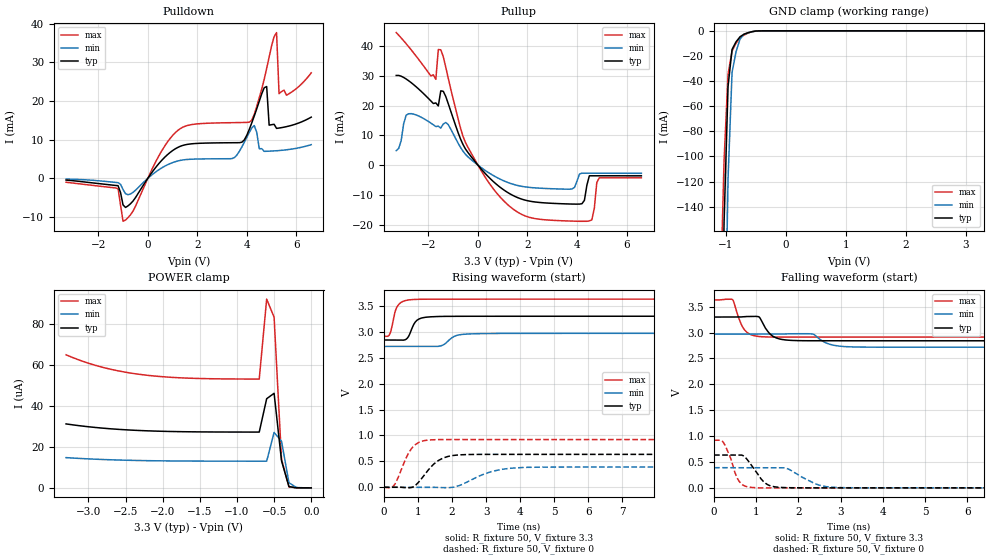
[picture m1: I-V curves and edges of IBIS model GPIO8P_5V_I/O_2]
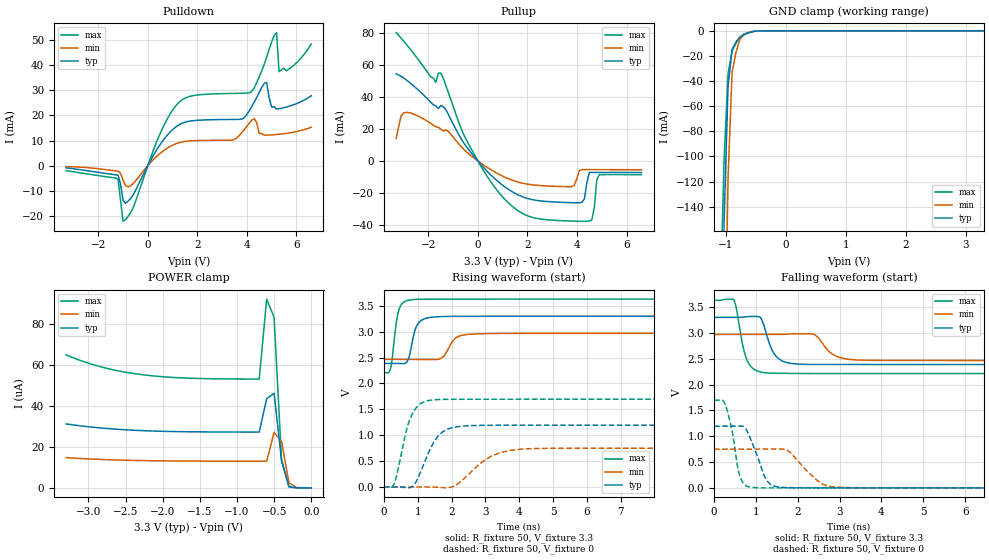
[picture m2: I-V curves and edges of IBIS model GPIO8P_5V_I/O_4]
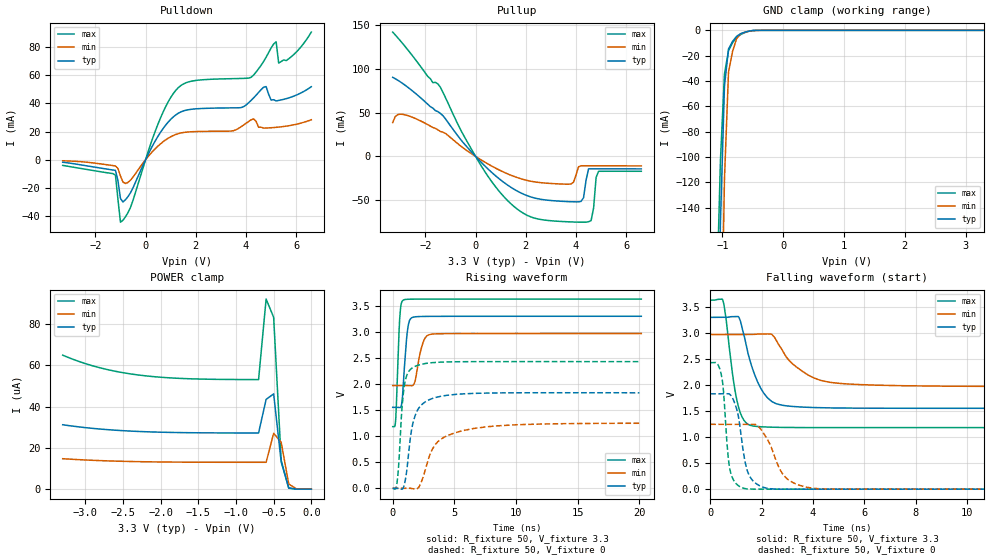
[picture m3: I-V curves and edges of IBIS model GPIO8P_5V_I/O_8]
[IBIS ver]   4.2
[File name]   tm4c123gh6pz_100qfp_v0p0.ibs
[File Rev]   v0p0
[Date]   Oct 16, 2013
[Source]   simulation
[Notes]   IBIS models for 100qfp package with updated GPIO models
[Disclaimer] Please be aware that in the absence of a written agreement,
   Texas Instruments (TI) assumes no liability for: 1) the
   accuracy of the IBIS models provided to your company, 2) the
   proper functioning of these IBIS models in your design or for
   any resulting applications, or; 3) infringement of patents,
   copyrights, or intellectual property rights resulting from
   your use of these IBIS models. TI provides IBIS models as a
   service to our customers and therefore reserves the right to
   limit distribution of the IBIS models.
   This preliminary model does not contain all of the possible pad
   models for each of the pad types.  The most commonly used modes
   have been provided and the next update will include all of the
   pad model combinations.
   The only missing model that needs to be highlighted is the
   model for the USB D+ and D- GPIOs.  Currently only the USB
   functionality is provided on the D+ and D- pins.  Customers
   needing to model the PGIOs associated with these pins should
   check for a newer model.
[Copyright]   Property of Texas Instruments Incorporated. Unauthorized
   reproduction and/or distribution is strictly prohibited. This
   product is protected under copyright law and trade secret law
   as an unpublished work. Copyright (C) 2013, Texas Instruments
   Incorporated, all rights reserved. These commodities are under
   the U.S. Government distribution license control. As such,
   they are not to be re-exported without the prior approval of
   the U.S. Department of Commerce.
|   Component TM4C123GH6PZ
[Component]   TM4C123GH6PZ
[Manufacturer]   Texas Instruments Inc.
[Package]
| 100-pin QFP
| variable   typ   min   max
R_Pkg   2.47E-01   2.19E-01   2.77E-01
L_pkg   5.75E-09   4.69E-09   6.71E-09
C_pkg   1.41E-12   1.29E-12   1.57E-12
[Pin]   signal_name   model_name   R_pin   L_pin   C_pin
1   PD0   GPIO8P_5V   2.73E-01   6.66E-09   1.34E-12
2   PD1   GPIO8P_5V   2.66E-01   6.52E-09   1.54E-12
3   PD2   GPIO8P_5V   2.54E-01   6.05E-09   1.51E-12
4   PD3   GPIO8P_5V   2.44E-01   5.86E-09   1.46E-12
5   VDD   POWER
6   GND   GND
7   VDDA   POWER
8   VREFAP   NC
9   VREFAM   NC
10   GNDA   GND
11   PJ2   GPIO8P_5V   2.19E-01   5.14E-09   1.32E-12
12   PE3   GPIO8P_5V   2.19E-01   5.16E-09   1.33E-12
13   PE2   GPIO8P_5V   2.19E-01   5.11E-09   1.34E-12
14   PE1   GPIO8P_5V   2.22E-01   5.08E-09   1.34E-12
15   PE0   GPIO8P_5V   2.25E-01   5.15E-09   1.33E-12
16   PH0   GPIO8P_5V   2.27E-01   5.31E-09   1.33E-12
17   PH1   GPIO8P_5V   2.32E-01   5.46E-09   1.37E-12
18   PH2   GPIO8P_5V   2.39E-01   5.53E-09   1.38E-12
19   PH3   GPIO8P_5V   2.48E-01   5.77E-09   1.38E-12
20   VDD   POWER
21   GND   GND
22   PC7   GPIO8P_5V   2.44E-01   5.93E-09   1.44E-12
23   PC6   GPIO8P_5V   2.54E-01   6.17E-09   1.50E-12
24   PC5   GPIO8P_5V   2.67E-01   6.47E-09   1.53E-12
25   PC4   GPIO8P_5V   2.74E-01   6.61E-09   1.32E-12
26   PA0_U0Rx   GPIO8P_5V   2.76E-01   6.71E-09   1.34E-12
27   PA1_U0Tx   GPIO8P_5V   2.70E-01   6.39E-09   1.55E-12
28   PA2_SSI0Clk   GPIO8P_5V   2.60E-01   6.25E-09   1.53E-12
29   PA3_SSI0Fss   GPIO8P_5V   2.52E-01   5.95E-09   1.51E-12
30   PA4_SSI0Rx   GPIO8P_5V   2.45E-01   5.72E-09   1.49E-12
31   PA5_SSI0Tx   GPIO8P_5V   2.41E-01   5.69E-09   1.46E-12
32   VDD   POWER
33   GND   GND
34   PA6   GPIO8P_5V   2.37E-01   5.51E-09   1.38E-12
35   PA7   GPIO8P_5V   2.38E-01   5.45E-09   1.37E-12
36   PF6   GPIO8P_5V   2.40E-01   5.41E-09   1.35E-12
37   PF5   GPIO8P_5V   2.43E-01   4.69E-09   1.30E-12
38   VDDC   POWER
39   PF4   GPIO8P_5V   2.44E-01   4.77E-09   1.31E-12
40   PF0   GPIO8P_5V   2.41E-01   5.42E-09   1.36E-12
41   PF1   GPIO8P_5V   2.38E-01   5.38E-09   1.37E-12
42   PF2   GPIO8P_5V   2.38E-01   5.50E-09   1.39E-12
43   PF3   GPIO8P_5V   2.39E-01   5.50E-09   1.40E-12
44   VDD   POWER
45   GND   GND
46   PK3   GPIO8P_5V   2.47E-01   5.79E-09   1.49E-12
47   PK2   GPIO8P_5V   2.54E-01   5.97E-09   1.51E-12
48   PK1   GPIO8P_5V   2.62E-01   6.12E-09   1.53E-12
49   PK0   GPIO8P_5V   2.72E-01   6.38E-09   1.55E-12
50   WAKE_n   RST_WAKE_INPUT  2.77E-01   6.58E-09   1.34E-12
51   HIB_n   HIB_OUTPUT   2.74E-01   6.58E-09   1.32E-12
52   XOSC0   NC
53   GNDX   GND
54   XOSC1   NC
55   VBAT   POWER
56   VDD   POWER
57   GND   GND
58   PF7   GPIO8P_5V   2.43E-01   5.77E-09   1.35E-12
59   PG3   GPIO8P_5V   2.36E-01   5.58E-09   1.36E-12
60   PG2   GPIO8P_5V   2.30E-01   5.33E-09   1.36E-12
61   PG1   GPIO8P_5V   2.24E-01   5.27E-09   1.35E-12
62   PG0   GPIO8P_5V   2.22E-01   5.12E-09   1.34E-12
63   RST_n   RST_WAKE_INPUT  2.19E-01   5.08E-09   1.34E-12
64   GND   GND
65   OSC0   NC
66   OSC1   NC
67   VDD   POWER
68   PJ0   USB_PHY_DM   2.32E-01   5.46E-09   1.37E-12
69   PJ1   USB_PHY_DP   2.34E-01   5.62E-09   1.39E-12
70   PB0_USB0ID   GPIO8P_5V   2.42E-01   5.80E-09   1.46E-12
71   PB1_USB0VBUS   GPIO8P_5V   2.49E-01   5.99E-09   1.48E-12
72   PB2_I2C0SCL   GPIO8P_5V   2.61E-01   6.31E-09   1.50E-12
73   PB3_I2C0SDA   GPIO8P_5V   2.73E-01   6.58E-09   1.50E-12
74   PG4   GPIO8P_5V   2.68E-01   6.56E-09   1.47E-12
75   PG5   GPIO8P_5V   2.76E-01   6.68E-09   1.29E-12
76   PH7   GPIO8P_5V   2.77E-01   6.60E-09   1.33E-12
77   PH6   GPIO8P_5V   2.71E-01   6.40E-09   1.54E-12
78   PH5   GPIO8P_5V   2.61E-01   6.16E-09   1.52E-12
79   PH4   GPIO8P_5V   2.52E-01   5.96E-09   1.50E-12
80   VDD   POWER
81   GND   GND
82   PC3_TDO_SWO   GPIO8P_5V   2.40E-01   5.50E-09   1.39E-12
83   PC2_TDI   GPIO8P_5V   2.37E-01   5.58E-09   1.38E-12
84   PC1_TMS_SWDIO  GPIO8P_5V   2.36E-01   5.44E-09   1.35E-12
85   PC0_TCK_SWCLK  GPIO8P_5V   2.36E-01   4.75E-09   1.31E-12
86   VDDC   POWER
87   PG6   GPIO8P_5V   2.43E-01   4.73E-09   1.33E-12
88   PG7   GPIO8P_5V   2.37E-01   5.35E-09   1.33E-12
89   PE6   GPIO8P_5V   2.40E-01   5.44E-09   1.36E-12
90   PE7   GPIO8P_5V   2.37E-01   5.38E-09   1.40E-12
91   PB5   GPIO8P_5V   2.35E-01   5.40E-09   1.42E-12
92   PB4   GPIO8P_5V   2.36E-01   4.85E-09   1.45E-12
93   VDD   POWER
94   GND   GND
95   PE4   GPIO8P_5V   2.40E-01   4.77E-09   1.52E-12
96   PE5   GPIO8P_5V   2.45E-01   5.74E-09   1.53E-12
97   PD4   GPIO8P_5V   2.52E-01   5.95E-09   1.54E-12
98   PD5   GPIO8P_5V   2.60E-01   6.23E-09   1.55E-12
99   PD6   GPIO8P_5V   2.70E-01   6.41E-09   1.57E-12
100   PD7   GPIO8P_5V   2.76E-01   6.59E-09   1.35E-12
[Model Selector] GPIO8P_5V
GPIO8P_5V_I/O_2   2mA Output Buffer
GPIO8P_5V_I/O_4   4mA Output Buffer
GPIO8P_5V_I/O_8S   8mA Output Buffer with Slew Rate Control
GPIO8P_5V_I/O_8   8mA Output Buffer
GPIO8P_5V_I_WPU_2   2mA Input with Pull-Up
GPIO8P_5V_I_WPD_2   2mA Input with Pull-Down
GPIO8P_5V_I/O_OD_2   2mA Output Buffer with Open Drain
GPIO8P_5V_I/O_OD_4   4mA Output Buffer with Open Drain
GPIO8P_5V_I/O_OD_8S   8mA Output Buffer with Open Drain and Slew Rate Control
GPIO8P_5V_I/O_OD_8   8mA Output Buffer with Open Drain
[Model Selector] RST_WAKE_INPUT
RST_WAKE_IN   Input Model for the WAKE_n Pin
[Model Selector] HIB_OUTPUT
HIBERNATE_OUTPUT   Output Buffer for the HIB_n Pin
[Model Selector] USB_PHY_DP
fsdp_tx   Full Speed transmitter--12Mbps
lsdp_50pf_tx   Low speed transmitter--1.5Mbps driving 50pF cap load
lsdp_200pf_tx   Low speed transmitter--1.5Mbps driving 200pF cap load
lsdp_400pf_tx   Low speed transmitter--1.5Mbps driving 400pF cap load
lsdp_600pf_tx   Low speed transmitter--1.5Mbps driving 600pF cap load
fsdp_rx   Recieve mode--Open circuit during fs/ls recieve mode
[Model Selector] USB_PHY_DM
fsdm_tx   Full Speed transmitter--12Mbps
lsdm_50pf_tx   Low speed transmitter--1.5Mbps driving 50pF cap load
lsdm_200pf_tx   Low speed transmitter--1.5Mbps driving 200pF cap load
lsdm_400pf_tx   Low speed transmitter--1.5Mbps driving 400pF cap load
lsdm_600pf_tx 	 Low speed transmitter--1.5Mbps driving 600pF cap load
fsdm_rx   Recieve mode--Open circuit during fs/ls recieve mode
| Models and submodels in the file (24): GPIO8P_5V_I/O_2 (I/O), GPIO8P_5V_I/O_4 (I/O), GPIO8P_5V_I/O_8S (I/O), GPIO8P_5V_I/O_8 (I/O), GPIO8P_5V_I_WPU_2 (Input), GPIO8P_5V_I_WPD_2 (Input), GPIO8P_5V_I/O_OD_2 (I/O_open_drain), GPIO8P_5V_I/O_OD_4 (I/O_open_drain), GPIO8P_5V_I/O_OD_8S (I/O_open_drain), GPIO8P_5V_I/O_OD_8 (I/O_open_drain), RST_WAKE_IN (Input), HIBERNATE_OUTPUT (Output), fsdp_tx (3-state), lsdp_50pf_tx (3-state), lsdp_200pf_tx (3-state), lsdp_400pf_tx (3-state), lsdp_600pf_tx (3-state), fsdp_rx (Input), fsdm_tx (3-state), lsdm_50pf_tx (3-state), lsdm_200pf_tx (3-state), lsdm_400pf_tx (3-state), lsdm_600pf_tx (3-state), fsdm_rx (Input)
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|   Model Cell GPIO8P_5V_I/O_2
[Model]   GPIO8P_5V_I/O_2
Model_type   I/O
Polarity   Non-Inverting
Enable   Active-Low
Vinl =  0.8
Vinh =  2
Cref =  15.0000pF
Rref =  100.0000M
Vref =  0V
Vmeas =  1.65
C_comp   4.711578p   4.034737p   5.423069p
[Model Spec]
Vinl   0.8   0.8   0.8
Vinh   2   2   2
[Temperature Range]   25   125   -40
[Voltage Range]   3.3   2.97   3.63
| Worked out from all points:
|   slope of the pulldown table from 0 to 0.495 V, typ, clamps not added: 118 ohm
|   slope of the pullup table from 0 to 0.495 V, typ, clamps not added: 109 ohm
|   GND clamp passes 1 mA (typ) near -0.59 V on its own axis
|   rising waveform, R_fixture 50, V_fixture 3.3: 20-80 % time 209ps typ, 304ps min, 170ps max; typ from 2.84 V to 3.3 V
|   rising waveform, R_fixture 50, V_fixture 0: 20-80 % time 527ps typ, 844ps min, 384ps max; typ from 0 V to 0.634 V
|   falling waveform, R_fixture 50, V_fixture 3.3: 20-80 % time 252ps typ, 337ps min, 213ps max; typ from 3.3 V to 2.84 V
|   falling waveform, R_fixture 50, V_fixture 0: 20-80 % time 342ps typ, 530ps min, 243ps max; typ from 0.634 V to 0 V
| Nom Voltages:
|   VDDC=1.2, VDD=3.3, GND=0
| Min Voltages:
|   VDDC=1.08, VDD=2.97, GND=0
| Max Voltages:
|   VDDC=1.32, VDD=3.63, GND=0
[POWER_clamp]
|   voltage   I(typ)   I(min)   I(max)
-3.3V     31.22uA    14.76uA    64.95uA
-3.1V     30.25uA    14.33uA    62.09uA
-2.8V     29.13uA    13.84uA    58.77uA
-2.3V     27.98uA    13.34uA    55.36uA
-1.7V     27.4uA     13.1uA     53.62uA
-700mV    27.24uA    13.03uA    53.12uA
-600mV    43.52uA    13.03uA    92.14uA
-500mV    46.16uA    27.05uA    83.3uA
-400mV    13.21uA    22.74uA    13.98uA
-300mV    630.7nA    2.501uA    480.9nA
-200mV    23.21nA    190.8nA    10.65nA
0V        660.4pA    10.19nA    564.9pA
[Pulldown]
|   voltage   I(typ)   I(min)   I(max)
-3.3V     -450.7uA   -192.2uA   -1.006mA
-1.2V     -1.893mA   -1.109mA   -2.697mA
-1V       -6.866mA   -2.892mA   -11.1mA
1.2V      7.958mA    4.478mA    12.33mA
3.5V      9.211mA    5.381mA    14.4mA
4.2V      14.36mA    13.04mA    15.06mA
4.5V      19.92mA    7.668mA    20.83mA
4.8V      23.73mA    7.004mA    28.42mA
4.9V      13.75mA    7.03mA     31.35mA
5.2V      12.91mA    7.14mA     37.68mA
5.3V      13mA       7.19mA     21.9mA
6.6V      15.82mA    8.714mA    27.27mA
[Pullup]
|   voltage   I(typ)   I(min)   I(max)
-3.3V     30.16mA    4.863mA    44.59mA
-2.9V     28.98mA    16.78mA    40.86mA
-1.7V     20.92mA    12.98mA    28.86mA
-1.6V     19.91mA    13.09mA    38.88mA
-1.5V     24.98mA    12.47mA    38.79mA
-500mV    5.386mA    3.597mA    7.551mA
1.6V      -10.92mA   -6.844mA   -15.8mA
3.8V      -13.1mA    -8.018mA   -18.83mA
4.2V      -12.99mA   -2.721mA   -18.9mA
4.5V      -3.591mA   -2.724mA   -18.76mA
4.9V      -3.59mA    -2.729mA   -4.279mA
6.6V      -3.606mA   -2.757mA   -4.278mA
[GND_clamp]
|   voltage   I(typ)   I(min)   I(max)
-3.3V     -16.3A     -15.26A    -17.13A
-1.1V     -340.4mA   -570.5mA   -222.8mA
-1.033V   -152.7mA   -296.8mA   -103.3mA
-966.7mV  -44.18mA   -117.7mA   -34.4mA
-900mV    -14.77mA   -33.12mA   -16.14mA
-833.3mV  -8.752mA   -16.68mA   -9.833mA
-766.7mV  -4.716mA   -6.551mA   -5.563mA
-700mV    -2.657mA   -2.741mA   -3.333mA
-566.7mV  -672.8uA   -727.2uA   -724.4uA
-433.3mV  -51.87uA   -90.8uA    -37.79uA
3.3V      660.4pA    5.308uA    422.7pA
[Ramp]
| variable   typ   min   max
dV/dt_f 0.28269897/0.25386606n 0.15654957/0.33829046n 0.43992818/0.21519855n
dV/dt_r 0.38699946/0.53401128n 0.23880101/0.85366195n 0.55927105/0.38819382n
R_load = 50
[Rising Waveform]
R_fixture = 50
V_fixture = 3.3
V_fixture_min = 2.97
V_fixture_max = 3.63
|   time   V(typ)   V(min)   V(max)
0s        2.841V     2.717V     2.912V
178.1ps   2.841V     2.717V     2.965V
341.5ps   2.841V     2.717V     3.419V
428.4ps   2.841V     2.717V     3.523V
687.2ps   2.877V     2.717V     3.61V
833.7ps   3.083V     2.717V     3.622V
1.166ns   3.274V     2.717V     3.628V
2.143ns   3.299V     2.931V     3.63V
2.818ns   3.299V     2.964V     3.63V
20.12ns   3.3V       2.97V      3.63V
[Rising Waveform]
R_fixture = 50
V_fixture = 0
V_fixture_min = 0
V_fixture_max = 0
|   time   V(typ)   V(min)   V(max)
0s        0V         0V         0V
320.1ps   0V         0V         57.85mV
634.7ps   -8.112mV   0V         543.5mV
833.3ps   0V         0V         764.8mV
1.337ns   360.6mV    0V         913.4mV
1.604ns   518.1mV    -4.493mV   919.6mV
2.025ns   613mV      0V         920.5mV
3.179ns   634.6mV    306.6mV    919.8mV
4.221ns   634.3mV    384.5mV    919.7mV
20.01ns   634.3mV    389.8mV    919.8mV
[Falling Waveform]
R_fixture = 50
V_fixture = 3.3
V_fixture_min = 2.97
V_fixture_max = 3.63
|   time   V(typ)   V(min)   V(max)
0s        3.3V       2.97V      3.63V
436.2ps   3.3V       2.97V      3.639V
720.2ps   3.308V     2.97V      3.054V
1.059ns   3.305V     2.97V      2.925V
1.179ns   3.141V     2.97V      2.917V
1.464ns   2.899V     2.97V      2.913V
2.039ns   2.843V     2.978V     2.913V
2.834ns   2.842V     2.755V     2.913V
3.318ns   2.841V     2.722V     2.913V
20.12ns   2.841V     2.717V     2.913V
[Falling Waveform]
R_fixture = 50
V_fixture = 0
V_fixture_min = 0
V_fixture_max = 0
|   time   V(typ)   V(min)   V(max)
0s        634.3mV    389.8mV    919.8mV
229.2ps   634.3mV    389.8mV    866.6mV
521.5ps   634.1mV    389.8mV    237.1mV
636.8ps   634.8mV    389.8mV    84.64mV
1.041ns   261.6mV    389.8mV    0V
1.409ns   23.56mV    389.7mV    0V
1.746ns   3.625mV    368.6mV    0V
2.48ns    0V         56.31mV    0V
3.006ns   0V         5.108mV    0V
20.01ns   0V         0V         0V
|   Model Cell GPIO8P_5V_I/O_4
[Model]   GPIO8P_5V_I/O_4
Model_type   I/O
Polarity   Non-Inverting
Enable   Active-Low
Vinl =  0.8
Vinh =  2
Cref =  15.0000pF
Rref =  100.0000M
Vref =  0V
Vmeas =  1.65
C_comp   4.711578p   4.034737p   5.423069p
[Model Spec]
Vinl   0.8   0.8   0.8
Vinh   2   2   2
[Temperature Range]   25   125   -40
[Voltage Range]   3.3   2.97   3.63
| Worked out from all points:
|   slope of the pulldown table from 0 to 0.495 V, typ, clamps not added: 59.3 ohm
|   slope of the pullup table from 0 to 0.495 V, typ, clamps not added: 59.2 ohm
|   GND clamp passes 1 mA (typ) near -0.59 V on its own axis
|   rising waveform, R_fixture 50, V_fixture 3.3: 20-80 % time 208ps typ, 290ps min, 166ps max; typ from 2.39 V to 3.3 V
|   rising waveform, R_fixture 50, V_fixture 0: 20-80 % time 516ps typ, 844ps min, 381ps max; typ from 0 V to 1.2 V
|   falling waveform, R_fixture 50, V_fixture 3.3: 20-80 % time 259ps typ, 347ps min, 216ps max; typ from 3.3 V to 2.39 V
|   falling waveform, R_fixture 50, V_fixture 0: 20-80 % time 329ps typ, 535ps min, 221ps max; typ from 1.2 V to 0 V
| Nom Voltages:
|   VDDC=1.2, VDD=3.3, GND=0
| Min Voltages:
|   VDDC=1.08, VDD=2.97, GND=0
| Max Voltages:
|   VDDC=1.32, VDD=3.63, GND=0
[POWER_clamp]
|   voltage   I(typ)   I(min)   I(max)
-3.3V     31.22uA    14.76uA    64.95uA
-3.1V     30.25uA    14.33uA    62.09uA
-2.8V     29.13uA    13.84uA    58.77uA
-2.3V     27.98uA    13.34uA    55.36uA
-1.7V     27.4uA     13.1uA     53.62uA
-700mV    27.24uA    13.03uA    53.12uA
-600mV    43.52uA    13.03uA    92.14uA
-500mV    46.16uA    27.05uA    83.3uA
-400mV    13.21uA    22.74uA    13.98uA
-300mV    630.7nA    2.501uA    480.9nA
-200mV    23.21nA    190.8nA    10.65nA
0V        660.4pA    10.19nA    564.9pA
[Pulldown]
|   voltage   I(typ)   I(min)   I(max)
-3.3V     -901.6uA   -384.4uA   -2.013mA
-1.2V     -3.786mA   -2.218mA   -5.418mA
-1V       -13.75mA   -5.79mA    -22.19mA
-700mV    -13.13mA   -8.08mA    -18.83mA
1.3V      16.5mA     9.253mA    25.59mA
3.5V      18.42mA    10.46mA    28.8mA
4.2V      23.61mA    18.14mA    29.55mA
4.8V      33.14mA    12.18mA    43.24mA
5V        23.36mA    12.28mA    49.33mA
5.2V      22.53mA    12.43mA    53.05mA
5.3V      22.7mA     12.52mA    37.48mA
6.6V      27.85mA    15.27mA    48.43mA
[Pullup]
|   voltage   I(typ)   I(min)   I(max)
-3.3V     54.59mA    14.22mA    80.39mA
-3.1V     52.96mA    28.24mA    76.9mA
-2.6V     47.05mA    29.37mA    67.36mA
-1.7V     34.57mA    21.42mA    49.25mA
-1.5V     34.64mA    19.97mA    55.03mA
100mV     -1.815mA   -1.128mA   -2.736mA
1.8V      -22.4mA    -13.91mA   -32.86mA
3.8V      -26.14mA   -15.97mA   -37.63mA
4.2V      -25.93mA   -5.421mA   -37.77mA
4.5V      -7.168mA   -5.427mA   -37.49mA
4.9V      -7.166mA   -5.439mA   -8.552mA
6.6V      -7.2mA     -5.497mA   -8.551mA
[GND_clamp]
|   voltage   I(typ)   I(min)   I(max)
-3.3V     -16.3A     -15.26A    -17.13A
-1.1V     -340.4mA   -570.5mA   -222.8mA
-1.033V   -152.7mA   -296.8mA   -103.3mA
-966.7mV  -44.18mA   -117.7mA   -34.4mA
-900mV    -14.77mA   -33.12mA   -16.14mA
-833.3mV  -8.752mA   -16.68mA   -9.833mA
-766.7mV  -4.716mA   -6.551mA   -5.563mA
-700mV    -2.657mA   -2.741mA   -3.333mA
-566.7mV  -672.8uA   -727.2uA   -724.4uA
-433.3mV  -51.87uA   -90.8uA    -37.79uA
3.3V      660.4pA    5.308uA    422.7pA
[Ramp]
| variable   typ   min   max
dV/dt_f  0.5587141/0.26045662n 0.31023858/0.352185n  0.86504244/0.21760119n
dV/dt_r 0.72667108/0.52198411n 0.45768162/0.8533017n   1.027789/0.38356156n
R_load = 50
[Rising Waveform]
R_fixture = 50
V_fixture = 3.3
V_fixture_min = 2.97
V_fixture_max = 3.63
|   time   V(typ)   V(min)   V(max)
0s        2.388V     2.466V     2.211V
198.6ps   2.388V     2.466V     2.297V
375ps     2.388V     2.466V     3.219V
457.4ps   2.387V     2.466V     3.451V
692.2ps   2.433V     2.466V     3.604V
849.4ps   2.842V     2.466V     3.621V
982.8ps   3.13V      2.466V     3.626V
1.222ns   3.257V     2.466V     3.629V
2.761ns   3.299V     2.959V     3.63V
20.01ns   3.3V       2.97V      3.63V
[Rising Waveform]
R_fixture = 50
V_fixture = 0
V_fixture_min = 0
V_fixture_max = 0
|   time   V(typ)   V(min)   V(max)
0s        0V         0V         0V
299.4ps   0V         0V         59.61mV
695.5ps   -16.31mV   0V         1.174V
860.4ps   17.92mV    0V         1.439V
1.44ns    827.9mV    0V         1.683V
1.727ns   1.062V     -12.61mV   1.693V
2.127ns   1.161V     33.95mV    1.695V
3.187ns   1.193V     597.4mV    1.696V
4.256ns   1.194V     739mV      1.696V
20.15ns   1.195V     748.9mV    1.696V
[Falling Waveform]
R_fixture = 50
V_fixture = 3.3
V_fixture_min = 2.97
V_fixture_max = 3.63
|   time   V(typ)   V(min)   V(max)
0s        3.3V       2.97V      3.63V
471.4ps   3.3V       2.97V      3.639V
817.4ps   3.316V     2.97V      2.422V
1.099ns   3.305V     2.97V      2.245V
1.273ns   2.918V     2.97V      2.224V
1.545ns   2.499V     2.97V      2.218V
2.126ns   2.392V     2.982V     2.214V
2.889ns   2.388V     2.56V      2.212V
3.475ns   2.388V     2.474V     2.212V
20.01ns   2.388V     2.466V     2.212V
[Falling Waveform]
R_fixture = 50
V_fixture = 0
V_fixture_min = 0
V_fixture_max = 0
|   time   V(typ)   V(min)   V(max)
0s        1.195V     748.8mV    1.697V
263ps     1.195V     748.8mV    1.625V
432ps     1.195V     748.8mV    1.1V
625.9ps   1.196V     748.8mV    202.3mV
899ps     892.7mV    748.8mV    9.985mV
1.272ns   130mV      748.8mV    0V
1.676ns   7.24mV     748.3mV    0V
2.497ns   0V         122.3mV    0V
3.021ns   0V         9.096mV    0V
20.15ns   0V         0V         0V
|   Model Cell GPIO8P_5V_I/O_8
[Model]   GPIO8P_5V_I/O_8
Model_type   I/O
Polarity   Non-Inverting
Enable   Active-Low
Vinl =  0.8
Vinh =  2
Cref =  15.0000pF
Rref =  100.0000M
Vref =  0V
Vmeas =  1.65
C_comp   4.711578p   4.034737p   5.423069p
[Model Spec]
Vinl   0.8   0.8   0.8
Vinh   2   2   2
[Temperature Range]   25   125   -40
[Voltage Range]   3.3   2.97   3.63
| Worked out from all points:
|   slope of the pulldown table from 0 to 0.495 V, typ, clamps not added: 29.7 ohm
|   slope of the pullup table from 0 to 0.495 V, typ, clamps not added: 34.2 ohm
|   GND clamp passes 1 mA (typ) near -0.59 V on its own axis
|   rising waveform, R_fixture 50, V_fixture 3.3: 20-80 % time 324ps typ, 517ps min, 232ps max; typ from 1.55 V to 3.3 V
|   rising waveform, R_fixture 50, V_fixture 0: 20-80 % time 786ps typ, 1.82ns min, 429ps max; typ from 0 V to 1.83 V
|   falling waveform, R_fixture 50, V_fixture 3.3: 20-80 % time 692ps typ, 1.23ns min, 406ps max; typ from 3.3 V to 1.55 V
|   falling waveform, R_fixture 50, V_fixture 0: 20-80 % time 366ps typ, 717ps min, 225ps max; typ from 1.83 V to 0 V
| Nom Voltages:
|   VDDC=1.2, VDD=3.3, GND=0
| Min Voltages:
|   VDDC=1.08, VDD=2.97, GND=0
| Max Voltages:
|   VDDC=1.32, VDD=3.63, GND=0
[POWER_clamp]
|   voltage   I(typ)   I(min)   I(max)
-3.3V     31.22uA    14.76uA    64.95uA
-3.1V     30.25uA    14.33uA    62.09uA
-2.8V     29.13uA    13.84uA    58.77uA
-2.3V     27.98uA    13.34uA    55.36uA
-1.7V     27.4uA     13.1uA     53.62uA
-700mV    27.24uA    13.03uA    53.12uA
-600mV    43.52uA    13.03uA    92.14uA
-500mV    46.16uA    27.05uA    83.3uA
-400mV    13.21uA    22.74uA    13.98uA
-300mV    630.7nA    2.501uA    480.9nA
-200mV    23.21nA    190.8nA    10.65nA
0V        660.3pA    10.19nA    564.9pA
[Pulldown]
|   voltage   I(typ)   I(min)   I(max)
-3.3V     -1.804mA   -768.9uA   -4.029mA
-1.2V     -7.576mA   -4.438mA   -10.94mA
-1V       -27.56mA   -11.61mA   -44.39mA
-700mV    -26.23mA   -16.15mA   -37.6mA
500mV     16.83mA    9.794mA    25.59mA
1.3V      32.99mA    18.5mA     51.14mA
3.5V      36.85mA    20.6mA     57.6mA
4.2V      42.1mA     28.33mA    58.55mA
4.8V      51.96mA    22.52mA    72.86mA
5.2V      41.77mA    23mA       83.78mA
5.3V      42.1mA     23.17mA    68.63mA
6.6V      51.87mA    28.39mA    90.67mA
[Pullup]
|   voltage   I(typ)   I(min)   I(max)
-3.3V     90.55mA    38.78mA    142.4mA
-2.4V     72.32mA    43.42mA    111.1mA
-1.4V     49.16mA    28.51mA    79.12mA
600mV     -17.27mA   -10.43mA   -27.2mA
2V        -44.4mA    -27.17mA   -66.73mA
3.8V      -51.96mA   -31.62mA   -75.08mA
4.2V      -51.61mA   -10.74mA   -75.41mA
4.5V      -14.27mA   -10.76mA   -74.89mA
4.6V      -14.27mA   -10.77mA   -73.6mA
4.8V      -14.27mA   -10.78mA   -23.97mA
4.9V      -14.27mA   -10.79mA   -17.08mA
6.6V      -14.35mA   -10.92mA   -17.08mA
[GND_clamp]
|   voltage   I(typ)   I(min)   I(max)
-3.3V     -16.3A     -15.26A    -17.13A
-1.1V     -340.4mA   -570.5mA   -222.8mA
-1.033V   -152.7mA   -296.8mA   -103.3mA
-966.7mV  -44.18mA   -117.7mA   -34.4mA
-900mV    -14.77mA   -33.12mA   -16.14mA
-833.3mV  -8.752mA   -16.68mA   -9.833mA
-766.7mV  -4.716mA   -6.551mA   -5.563mA
-700mV    -2.657mA   -2.741mA   -3.333mA
-566.7mV  -672.8uA   -727.2uA   -724.4uA
-433.3mV  -51.87uA   -90.8uA    -37.79uA
3.3V      660.3pA    5.308uA    422.7pA
[Ramp]
| variable   typ   min   max
dV/dt_f  1.0583429/0.69409355n 0.60650749/1.2284824n  1.4815153/0.407993n
dV/dt_r  1.1099303/0.78949909n 0.75855304/1.8220444n  1.4680093/0.43078817n
R_load = 50
[Rising Waveform]
R_fixture = 50
V_fixture = 3.3
V_fixture_min = 2.97
V_fixture_max = 3.63
|   time   V(typ)   V(min)   V(max)
0s        1.553V     1.971V     1.183V
228.9ps   1.553V     1.971V     1.278V
565.1ps   1.548V     1.971V     3.248V
738.6ps   1.634V     1.971V     3.573V
859.6ps   1.992V     1.971V     3.61V
1.22ns    3.068V     1.971V     3.626V
1.67ns    3.283V     1.982V     3.628V
2.46ns    3.297V     2.795V     3.629V
3.093ns   3.298V     2.955V     3.629V
20.17ns   3.3V       2.97V      3.63V
[Rising Waveform]
R_fixture = 50
V_fixture = 0
V_fixture_min = 0
V_fixture_max = 0
|   time   V(typ)   V(min)   V(max)
0s        0V         0V         0V
364.1ps   0V         0V         131.1mV
754.4ps   -15.59mV   0V         1.54V
971.2ps   95.88mV    0V         2.009V
1.493ns   1.075V     -2.242mV   2.293V
1.765ns   1.356V     -14.08mV   2.334V
2.211ns   1.569V     59.87mV    2.372V
3.451ns   1.74V      839.2mV    2.414V
5.161ns   1.803V     1.072V     2.427V
20.01ns   1.831V     1.248V     2.43V
[Falling Waveform]
R_fixture = 50
V_fixture = 3.3
V_fixture_min = 2.97
V_fixture_max = 3.63
|   time   V(typ)   V(min)   V(max)
0s        3.3V       2.97V      3.63V
490.6ps   3.3V       2.97V      3.627V
1.062ns   3.316V     2.97V      1.651V
1.299ns   2.986V     2.97V      1.333V
1.561ns   2.445V     2.97V      1.226V
2.222ns   1.757V     2.982V     1.193V
3.023ns   1.597V     2.501V     1.185V
4.016ns   1.568V     2.141V     1.183V
5.4ns     1.557V     2.019V     1.182V
20.17ns   1.553V     1.971V     1.182V
[Falling Waveform]
R_fixture = 50
V_fixture = 0
V_fixture_min = 0
V_fixture_max = 0
|   time   V(typ)   V(min)   V(max)
0s        1.831V     1.246V     2.43V
451.2ps   1.831V     1.246V     2.146V
708.2ps   1.833V     1.246V     568.9mV
860.7ps   1.757V     1.246V     218.6mV
1.086ns   1.424V     1.246V     70.85mV
1.297ns   688.8mV    1.246V     16.52mV
1.907ns   69.1mV     1.188V     0V
2.916ns   0V         235.1mV    0V
4ns       0V         18.15mV    0V
20.01ns   0V         0V         0V
